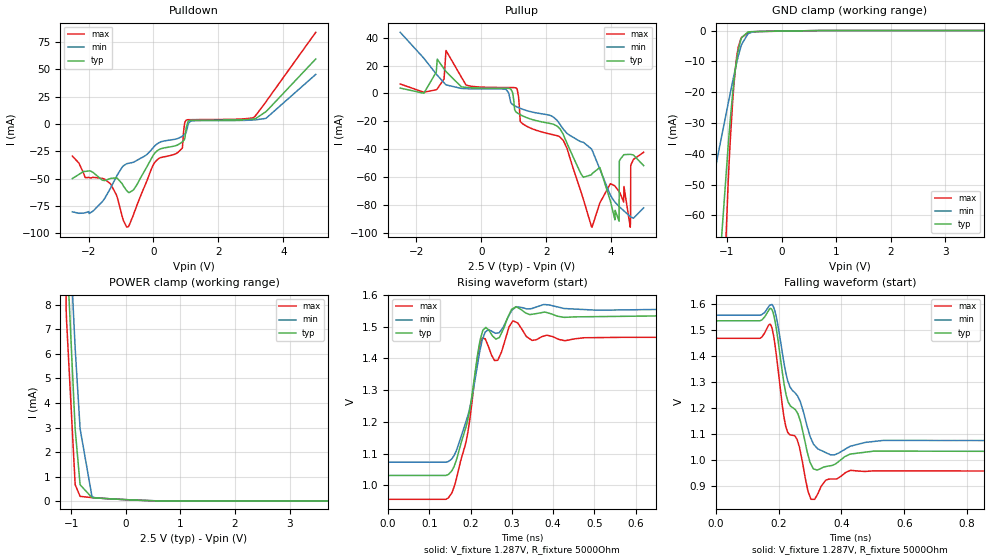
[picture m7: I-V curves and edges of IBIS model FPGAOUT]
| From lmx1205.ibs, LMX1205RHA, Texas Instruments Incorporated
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|   Model FPGAOUT
[Model]   FPGAOUT
Model_type   Output
Polarity   Non-Inverting
Vmeas = 1.25
Vref = 1.25
Cref = 2pF
Rref = 50
|   typ   min   max
C_comp   0.503pF   0.430pF   0.580pF
[Voltage Range]   2.5   2.4   2.6
[Temperature Range]   27   105   -40
[Pullup Reference]   2.5   2.4   2.6
[Pulldown Reference]   0   0   0
[Power Clamp Reference]   2.5   2.4   2.6
[GND Clamp Reference]   0   0   0
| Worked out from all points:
|   slope of the pulldown table from 0 to 0.375 V, typ, clamps not added: 56 ohm
|   slope of the pullup table from 0 to 0.375 V, typ, clamps not added: 4.59 kohm
|   GND clamp passes 1 mA (typ) near -0.65 V on its own axis
|   POWER clamp passes 1 mA (typ) near -0.85 V on its own axis
|   falling waveform, V_fixture 1.287V, R_fixture 5000Ohm: 20-80 % time 71.6ps typ, 76.6ps min, 67.4ps max; typ from 1.53 V to 1.03 V
|   rising waveform, V_fixture 1.287V, R_fixture 5000Ohm: 20-80 % time 43.2ps typ, 47.7ps min, 40.3ps max; typ from 1.03 V to 1.53 V
[Pulldown]
|   Voltage   I(typ)   I(min)   I(max)
-2.5V     -49.85mA   -80.22mA   -29.2mA
-2.103V   -43.27mA   -81.09mA   -49.01mA
-1.323V   -49.68mA   -58.59mA   -54.72mA
-775mV    -62.38mA   -35.91mA   -93.83mA
42.5mV    -26.5mA    -19.9mA    -35mA
882.5mV   -16.43mA   -11.18mA   -22.18mA
950mV     -14.25mA   -9.664mA   -1.316mA
1.002V    -4.533mA   -7.852mA   3.476mA
1.167V    3.516mA    2.847mA    4.032mA
3.125V    4.799mA    3.837mA    6.936mA
3.462V    11.27mA    5.212mA    20.2mA
5V        59.53mA    45.41mA    83.9mA
[GND Clamp]
|   Voltage   I(typ)   I(min)   I(max)
-2.5V     -415.3mA   -207.5mA   -737.4mA
-1.502V   -164.3mA   -71.12mA   -318.1mA
-1.105V   -68.94mA   -35.09mA   -107.5mA
-977.5mV  -37.53mA   -23.72mA   -49.54mA
-940mV    -29.18mA   -20.43mA   -36.11mA
-895mV    -20.37mA   -16.53mA   -23.03mA
-850mV    -13.27mA   -12.76mA   -13.2mA
-820mV    -9.434mA   -10.38mA   -8.363mA
-790mV    -6.167mA   -8.157mA   -5.209mA
-730mV    -2.306mA   -4.48mA    -2.234mA
-617.5mV  -503.4uA   -1.145mA   -754.9uA
5V        0A         0A         0A
[Pullup]
|   Voltage   I(typ)   I(min)   I(max)
-2.5V     3.778mA    43.83mA    6.713mA
-1.36V    24.57mA    13.05mA    3.218mA
-1.09V    15.64mA    6.106mA    30.81mA
1.085V    -13.64mA   -9.575mA   3.645mA
1.212V    -15.48mA   -10.86mA   -20.55mA
2.533V    -30.02mA   -25.93mA   -34.2mA
3.41V     -57.62mA   -40.63mA   -96.03mA
4.242V    -91.82mA   -81.13mA   -70.37mA
4.25V     -48.62mA   -81.31mA   -70.66mA
4.588V    -43.76mA   -88.41mA   -96.04mA
4.603V    -43.78mA   -88.65mA   -51.5mA
5V        -51.85mA   -82.22mA   -42.26mA
[POWER Clamp]
|   Voltage   I(typ)   I(min)   I(max)
-2.5V     188.2mA    95.85mA    235.6mA
-1.097V   11.25mA    14.18mA    19.21mA
-1.09V    10.84mA    13.81mA    7.801mA
-1.083V   10.42mA    13.44mA    7.351mA
-925mV    2.921mA    6.22mA     668.4uA
-835mV    668.8uA    2.951mA    194.2uA
-617.5mV  140.6uA    181uA      143.3uA
-587.5mV  136uA      154.4uA    138.6uA
-10mV     61.39uA    63.22uA    60.22uA
807.5mV   2.988uA    3.134uA    3.017uA
5V        0A         0A         0A
[Ramp]
R_load = 5000
|   typ   min   max
dV/dt_r   0.301538/4.31999e-11   0.289498/4.9732e-11   0.306152/5.30735e-11
dV/dt_f   0.302032/7.15719e-11   0.289842/7.65268e-11   0.306802/6.7445e-11
[Falling Waveform]
V_fixture = 1.287V
V_fixture_min = 1.319V
V_fixture_max = 1.215V
R_fixture = 5000Ohm
C_fixture = 0F
|   Time   V(typ)   V(min)   V(max)
0s        1.535V     1.556V     1.467V
140ps     1.535V     1.556V     1.467V
175.8ps   1.581V     1.597V     1.517V
192ps     1.507V     1.551V     1.406V
222.3ps   1.257V     1.336V     1.129V
258.2ps   1.183V     1.248V     1.079V
302.6ps   983.2mV    1.082V     847.9mV
364.5ps   976.8mV    1.019V     925.8mV
428.9ps   1.022V     1.052V     959.2mV
1.27ns    1.031V     1.073V     956mV
[Rising Waveform]
V_fixture = 1.287V
V_fixture_min = 1.319V
V_fixture_max = 1.215V
R_fixture = 5000Ohm
C_fixture = 0F
|   Time   V(typ)   V(min)   V(max)
0s        1.032V     1.073V     956.4mV
146.3ps   1.035V     1.075V     961mV
161.1ps   1.064V     1.097V     999.1mV
189.9ps   1.189V     1.205V     1.143V
216.7ps   1.409V     1.38V      1.403V
228.4ps   1.482V     1.458V     1.464V
266ps     1.463V     1.48V      1.394V
302.6ps   1.557V     1.554V     1.518V
349.3ps   1.539V     1.557V     1.457V
1.27ns    1.534V     1.556V     1.467V
